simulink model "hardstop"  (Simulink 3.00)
settings: Solver=ode45  SolverMode=SingleTasking  StartTime=0.0  StopTime=2.0  RelTol=1e-6  AbsTol=1e-6

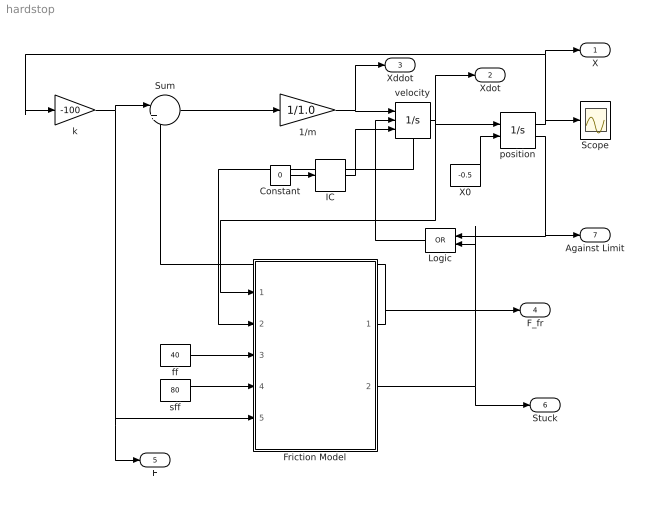
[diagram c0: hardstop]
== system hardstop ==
  1/m : Gain  Gain=1/1.0  SaturateOnIntegerOverflow=on
  Constant : Constant  Value=0
  Friction Model : Subsystem
  IC : InitialCondition  Value=100
  Logic : Logic  Orientation=left  Operator=OR  Inputs=2
  Scope : Scope
  Sum : Sum  Inputs=|+-  SaturateOnIntegerOverflow=on
  X0 : Constant  Value=-0.5
  ff : Constant  Value=40
  k : Gain  Gain=-100  SaturateOnIntegerOverflow=on
  position : Integrator  ExternalReset=none  InitialConditionSource=external  InitialCondition=0  LimitOutput=on  UpperSaturationLimit=5.5  LowerSaturationLimit=-3.5  ShowSaturationPort=on  ShowStatePort=off  AbsoluteTolerance=auto
  sff : Constant  Value=80
  velocity : Integrator  ExternalReset=rising  InitialConditionSource=external  InitialCondition=0  LimitOutput=off  UpperSaturationLimit=inf  LowerSaturationLimit=-inf  ShowSaturationPort=off  ShowStatePort=on  AbsoluteTolerance=auto
  X : Outport  Port=1  InitialOutput=0
  Xdot : Outport  Port=2  InitialOutput=0
  Xddot : Outport  Port=3  InitialOutput=0
  F_fr : Outport  Port=4  InitialOutput=0
  F : Outport  Port=5  InitialOutput=0
  Stuck : Outport  Port=6  InitialOutput=0
  Against Limit : Outport  Port=7  InitialOutput=0
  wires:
  position/1 -> Scope/1, k/1, X/1
  position/2 -> Against Limit/1, Logic/1
  Constant/1 -> IC/1
  X0/1 -> position/2
  Sum/1 -> 1/m/1
  IC/1 -> velocity/3
  velocity/1 -> Xdot/1, position/1, Friction Model/1(velocity)
  k/1 -> Sum/1, F/1, Friction Model/5(force)
  1/m/1 -> velocity/1, Xddot/1
  sff/1 -> Friction Model/4(static friction)
  ff/1 -> Friction Model/3(kinetic friction)
  Friction Model/2(Stuck) -> Stuck/1, Logic/2
  velocity/State -> Friction Model/2(velocity_stateport1)
  Logic/1 -> velocity/2
  Friction Model/1(F_fr) -> F_fr/1, Sum/2

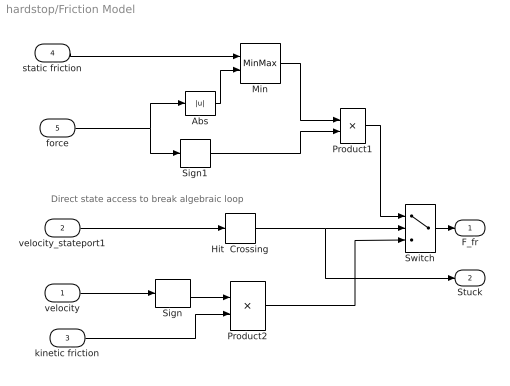
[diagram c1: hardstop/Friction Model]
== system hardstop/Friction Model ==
  note: Direct state access to break algebraic loop
  velocity : Inport  Port=1  PortWidth=-1  SampleTime=-1  DataType=auto
  velocity_stateport1 : Inport  Port=2  PortWidth=-1  SampleTime=-1  DataType=auto
  kinetic friction : Inport  Port=3  PortWidth=-1  SampleTime=-1  DataType=auto
  static friction : Inport  Port=4  PortWidth=-1  SampleTime=-1  DataType=auto
  force : Inport  Port=5  PortWidth=-1  SampleTime=-1  DataType=auto
  Abs : Abs
  Hit  Crossing : HitCross  HitCrossingOffset=0  HitCrossingDirection=either  ShowOutputPort=on
  Min : MinMax  Function=min  Inputs=2
  Product1 : Product  Inputs=2  SaturateOnIntegerOverflow=on
  Product2 : Product  Inputs=2  SaturateOnIntegerOverflow=on
  Sign : Signum
  Sign1 : Signum
  Switch : Switch  Threshold=0.5
  F_fr : Outport  Port=1  InitialOutput=0
  Stuck : Outport  Port=2  InitialOutput=0
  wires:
  Hit  Crossing/1 -> Stuck/1, Switch/2
  Product2/1 -> Switch/3
  kinetic friction/1 -> Product2/2
  Sign/1 -> Product2/1
  velocity/1 -> Sign/1
  Switch/1 -> F_fr/1
  velocity_stateport1/1 -> Hit  Crossing/1
  Product1/1 -> Switch/1
  force/1 -> Abs/1, Sign1/1
  Abs/1 -> Min/2
  static friction/1 -> Min/1
  Min/1 -> Product1/1
  Sign1/1 -> Product1/2
